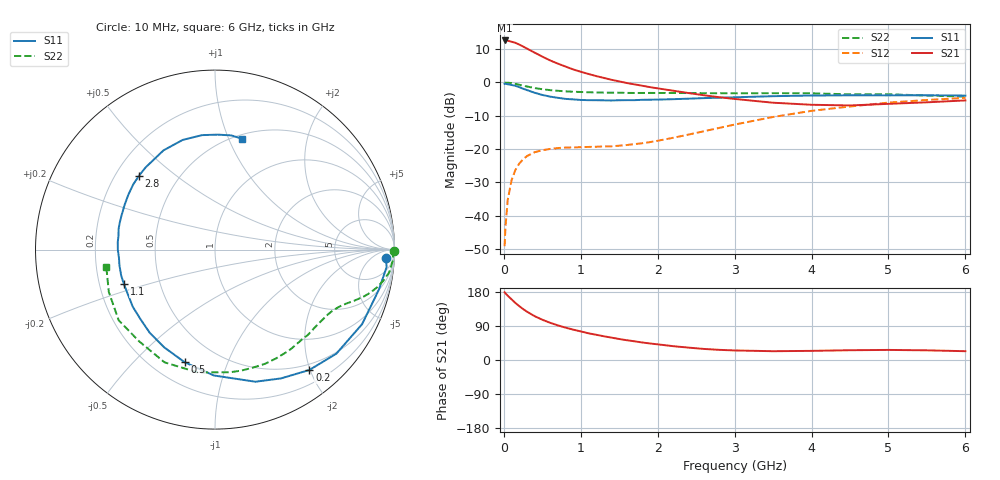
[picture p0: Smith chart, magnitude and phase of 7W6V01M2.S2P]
! Infineon Technologies  Discrete & RF Semiconductors
! BFS17W
! Si NPN RF Bipolar Junction Transistor in SOT323
! VCE = 6 V  IC = 1.2 mA
! Common Emitter S-Parameters:  August  1999
# GHz  S  MA  R  50
!  f  S11  S21  S12  S22
! GHz  MAG  ANG  MAG  ANG  MAG  ANG  MAG  ANG
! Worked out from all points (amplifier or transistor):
!   36 points, 10 MHz to 6 GHz, reference 50 ohm
!   highest |S21| = 12.6 dB at 10 MHz (marker M1)
!   |S21| within 3 dB of that: start of sweep to 347 MHz
!   unconditionally stable (mu >= 1): 1.001 GHz to 3.375 GHz; 3.849 GHz to end of sweep
!   at 250 MHz: K = 0.27, MSG = 16.9 dB, |S12| = -23.1 dB
!   at 1.4 GHz: K = 1.27, MAG = 6.9 dB, |S12| = -19.1 dB
!   at 6 GHz: K = 1.09, MAG = -2.2 dB, |S12| = -4.6 dB
!   S11 on the Smith chart (normalised r, x): 10 MHz: 21, -20; 200 MHz: 0.41, -1.99; 500 MHz: 0.33, -0.71; 1.1 GHz: 0.31, -0.17; 2.8 GHz: 0.30, +0.38; 6 GHz: 0.54, +1.12
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0.01  0.9519 -2.7  4.27 178.6  0.0035 87.4  0.9999 -0.3
0.02  0.9613 -5.8  4.27 176.0  0.0065 86.3  0.9924 -1.5
0.05  0.9398 -13.8  4.236 169.7  0.0172 82.6  0.9916 -3.8
0.1  0.9188 -26.9  4.089 160.2  0.034 74.9  0.9785 -7.5
0.15  0.8907 -40.6  3.935 150.6  0.0487 67.6  0.9516 -10.7
0.2  0.8523 -51.9  3.709 142.2  0.0606 62.6  0.9248 -13.3
0.25  0.8063 -62.9  3.468 134.5  0.0702 56.2  0.8965 -15.6
0.3  0.7697 -73.0  3.231 127.6  0.0786 52.1  0.8707 -17.4
0.4  0.7014 -90.5  2.804 115.7  0.0898 45.3  0.8258 -20.2
0.5  0.6502 -105.0  2.446 106.3  0.0962 40.8  0.7916 -22.3
0.6  0.6139 -117.4  2.146 98.3  0.1006 38.2  0.7679 -24.1
0.7  0.5892 -128.1  1.922 91.5  0.1037 36.6  0.7506 -25.9
0.9  0.5578 -145.3  1.573 80.2  0.106 35.4  0.7261 -29.7
1.1  0.5428 -159.1  1.342 70.5  0.1079 37.2  0.7132 -33.8
1.4  0.537 -175.0  1.097 59.0  0.1103 42.6  0.7039 -40.4
1.6  0.5434 175.5  0.981 52.1  0.1153 47.3  0.6973 -45.2
2.2  0.5616 153.9  0.753 36.5  0.1478 61.5  0.6953 -60.8
2.8  0.5907 135.7  0.601 26.8  0.2082 67.9  0.6901 -77.7
3.5  0.623 117.4  0.497 23.2  0.3038 66.1  0.6914 -97.9
4.5  0.6418 96.4  0.452 25.8  0.4359 53.9  0.6632 -129.5
5.5  0.6426 81.9  0.504 25.5  0.5462 40.3  0.637 -158.2
6  0.6359 76.5  0.538 23.2  0.5881 33.8  0.6132 -171.0
